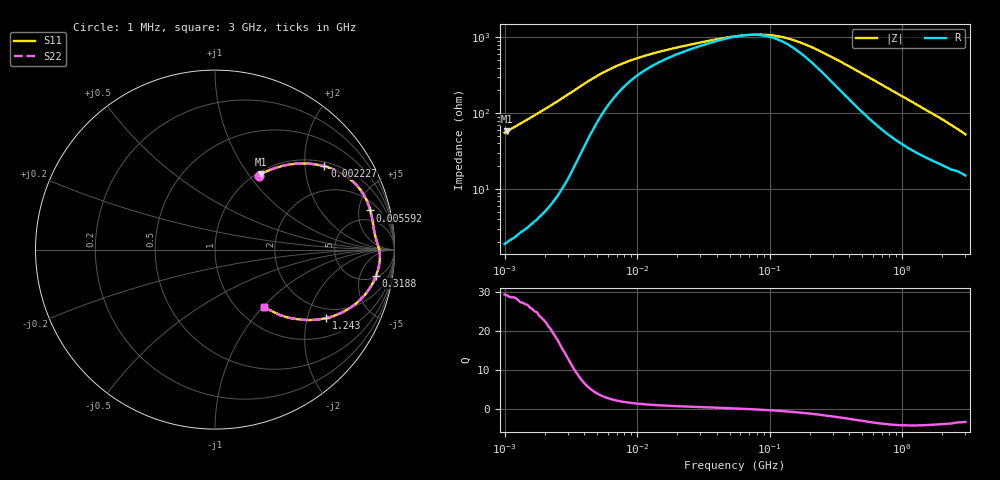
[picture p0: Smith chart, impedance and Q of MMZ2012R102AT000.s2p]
! S-parameter Generated by TDK Corporation
! Copyright(C) 2016 TDK Corporation.
! All Rights Reserved.
! TDK P/N: MMZ2012R102AT000 (Chip Beads)
! Property: |Z|=1000¶ at 100MHz
! Size(LxWxT): 2x1.25x0.85mm, 0.079x0.049x0.033inches
! Model Type: s2p (Touchstone File Format Version 1.0)
! Frequency: DC=Yes Start=1MHz Stop=3000MHz 202points Log-sweep
! Note: This model was converted from impedance.
! Model Generated on May. 16, 2016
! Hash(MD5):
! Port Assignments:
!  1 ---@@@--- 2
! Applicable Conditions:
!  Temperature = 25 degC
!  DC Bias Current = 0 A
!  Small Signal Operation
! Terms and conditions regarding TDK Simulation Models
! (1)This simulation model is being provided solely for informational purposes. Please refer to the specifications of the products in terms of detailed characteristics of such products.
! (2)In no event shall TDK Corporation of any of its subsidiaries be liable for any loss or damage arising, directly or indirectly,
!  From any information contained in this simulation model, including, but not limited to loss or damages arising from any inaccuracies, omissions or errors in connection with such information.
! (3)Any and all copyrights on this simulation model are owned by TDK Corporation.
!  Duplication or redistribution of this simulation model without prior written permission from TDK Corporation is prohibited.
! (4)This simulation model is subject to any modification or change without any prior notice.
! (5)Neither TDK Corporation nor any of its subsidiaries shall make any warranty, express or implied,
!  Including but not limited to the correctness, implied warranties of merchantability and fitness for a particular purpose with respect to this simulation models.
! (6)The use of this simulation model shall be deemed to have consented to the terms and conditions hereof.
# MHz S MA R 50
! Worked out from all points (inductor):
!   201 points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, 1 MHz to 3 GHz, reference 50 ohm
!   read as one part in series: L = 8.83 uH near 1.041 MHz
!   highest Q = 29.2 at 1.041 MHz (marker M1), where L = 8.82 uH
!   self-resonance near 67.1 MHz
!   S11 on the Smith chart (normalised r, x): 1 MHz: 1.04, +1.11; 2.227 MHz: 1.12, +2.52; 5.592 MHz: 3.10, +6.63; 318.8 MHz: 6, -9; 1.243 GHz: 1.62, -2.63; 3 GHz: 1.30, -1.01
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1  0.4783 59.5  0.8621 -28.6  0.8621 -28.6  0.4783 59.5
1.040844  0.4928 58.5  0.8534 -29.5  0.8534 -29.5  0.4928 58.5
1.553251  0.6422 47.9  0.7423 -39.9  0.7423 -39.9  0.6422 47.9
2.226959  0.7661 37.3  0.6065 -49.9  0.6065 -49.9  0.7661 37.3
3.067588  0.8469 27.8  0.4681 -57.6  0.4681 -57.6  0.8469 27.8
3.900413  0.8792 21.4  0.3685 -60.5  0.3685 -60.5  0.8792 21.4
5.592179  0.8923 14.2  0.2565 -58.3  0.2565 -58.3  0.8923 14.2
8.686058  0.8921 8.9  0.1821 -49.3  0.1821 -49.3  0.8921 8.9
14.61624  0.8948 5.4  0.1383 -37.8  0.1383 -37.8  0.8948 5.4
33.87922  0.9061 2.2  0.1009 -20.3  0.1009 -20.3  0.9061 2.2
54.77226  0.9127 0.7  0.08803 -7.0  0.08803 -7.0  0.9127 0.7
81.73662  0.9172 -0.7  0.08367 7.8  0.08367 7.8  0.9172 -0.7
108.1723  0.919 -1.8  0.08668 20.0  0.08668 20.0  0.919 -1.8
149.005  0.9197 -3.4  0.09867 33.8  0.09867 33.8  0.9197 -3.4
213.6344  0.9177 -5.7  0.1257 46.4  0.1257 46.4  0.9177 -5.7
318.8066  0.9097 -9.2  0.177 54.8  0.177 54.8  0.9097 -9.2
536.4635  0.8791 -15.7  0.2827 57.1  0.2827 57.1  0.8791 -15.7
800.5644  0.8266 -22.6  0.3957 53.3  0.3957 53.3  0.8266 -22.6
1243.477  0.7275 -31.6  0.5389 45.1  0.5389 45.1  0.7275 -31.6
1931.433  0.5869 -41.1  0.6777 34.7  0.6777 34.7  0.5869 -41.1
2359.433  0.5125 -45.3  0.7362 29.7  0.7362 29.7  0.5125 -45.3
3000  0.4188 -49.7  0.7957 23.7  0.7957 23.7  0.4188 -49.7
